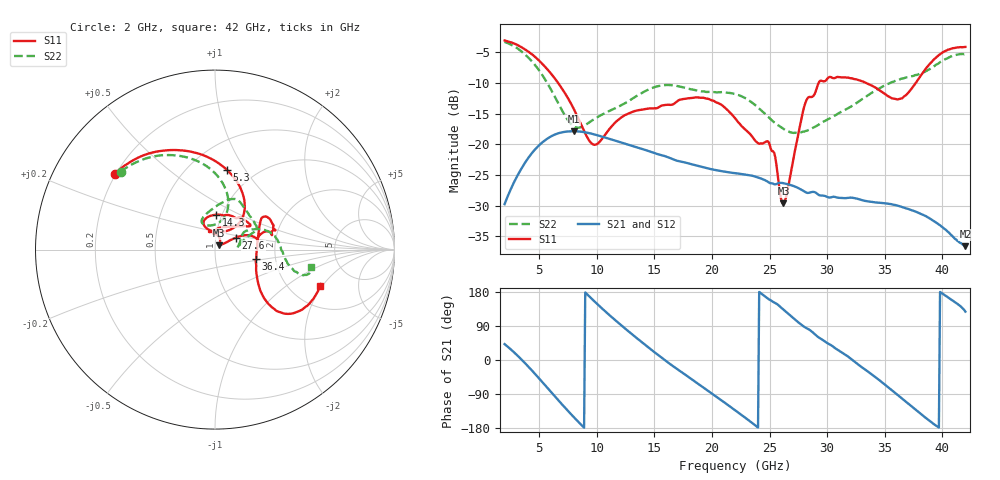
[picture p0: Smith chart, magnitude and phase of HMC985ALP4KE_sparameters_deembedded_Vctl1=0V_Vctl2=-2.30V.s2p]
!s2p File: Measurements: S11, S21, S12, S22
# GHz S dB R 50.0
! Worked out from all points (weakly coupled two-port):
!   401 points, 2 GHz to 42 GHz, reference 50 ohm
!   highest |S21| = -17.88 dB at 8 GHz (marker M1); lowest = -36.6 dB at 42 GHz (marker M2)
!   lowest |S11| = -29.6 dB at 26.2 GHz (marker M3), VSWR 1.07, Z = 52.3 + j2.46 ohm
!   |S11| at or under -10 dB: 6.642 GHz to 29.26 GHz (22.62 GHz wide, 126 % of centre); 33.37 GHz to 37.7 GHz (4.326 GHz wide, 12.2 % of centre)
!   |S22| runs from -18.2 to -3.3 dB; largest |S21 - S12| = 0.0005
!   S11 on the Smith chart (normalised r, x): 2 GHz: 0.20, +0.32; 5.3 GHz: 0.75, +0.83; 14.3 GHz: 0.94, +0.38; 27.6 GHz: 1.25, +0.17; 36.4 GHz: 1.58, -0.18; 42 GHz: 2.91, -1.91
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2  -3.09 142.8  -29.76 41.9  -29.75 42.0  -3.33 140.5
3.5  -4.23 115.8  -23.84 0.2  -23.85 0.1  -4.93 112.3
5.3  -6.95 81.5  -19.65 -59.2  -19.67 -59.3  -8.80 82.3
8  -14.22 47.8  -17.88 -150.6  -17.86 -150.6  -17.07 89.5
8.7  -17.04 52.4  -17.97 -172.5  -17.97 -172.5  -17.18 104.4
9.9  -20.06 87.9  -18.45 151.8  -18.45 151.8  -15.76 115.6
12.2  -15.54 112.2  -19.77 89.7  -19.75 89.7  -13.57 101.2
14.3  -14.22 88.4  -20.98 37.6  -20.96 37.6  -11.26 78.8
15.4  -13.94 73.3  -21.67 11.7  -21.69 11.6  -10.50 71.0
19.3  -12.44 34.1  -23.78 -73.5  -23.79 -73.5  -11.39 42.4
22  -15.74 52.3  -24.71 -132.3  -24.73 -132.4  -11.82 25.7
25  -20.01 98.7  -26.30 159.2  -26.27 159.3  -15.76 17.5
26.2  -29.63 45.3  -26.34 133.0  -26.38 133.0  -17.51 8.5
27.6  -17.37 29.8  -27.24 96.9  -27.24 96.9  -18.06 4.4
28.1  -13.30 20.9  -27.79 85.7  -27.82 85.7  -17.88 6.4
28.7  -12.27 13.0  -27.77 74.2  -27.75 74.1  -17.38 10.7
31  -9.05 23.3  -28.72 25.2  -28.70 25.2  -14.94 29.9
33.3  -9.94 34.2  -29.23 -25.3  -29.23 -25.2  -12.35 27.8
35.4  -12.27 12.1  -29.71 -74.5  -29.70 -74.5  -10.08 18.8
36.4  -12.58 -13.1  -30.16 -99.3  -30.18 -99.4  -9.34 12.9
39.5  -5.81 -43.4  -32.81 -174.2  -32.78 -174.1  -7.00 -14.0
42  -4.14 -19.0  -36.60 127.7  -36.59 127.5  -5.31 -10.5
